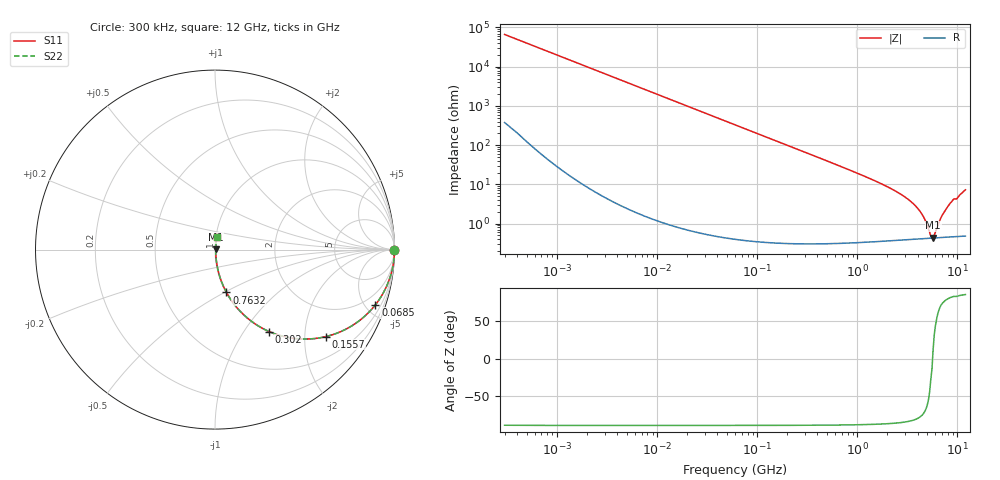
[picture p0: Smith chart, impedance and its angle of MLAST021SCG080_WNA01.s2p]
! MLAST021SCG080_WNA01  S-PARAMETER MODEL  ( General Type )
! Model Generated by TAIYO YUDEN Corporation (http://www.ty-top.com)
! Version 1.0
! TAIYO YUDEN Control No. 220901
! Copyright(c) 2022 TAIYO YUDEN CO.,LTD. All Rights Reserved.
! Product Description (link to TY-COMPAS)
! https://ds.yuden.co.jp/TYCOMPAS/or/detail?pn=MLAST021SCG080CWNA01&u=M
! Products Name : Multilayer Ceramic Capacitors
! Characteristics :
!  Capacitance : 8 pF , Rated Voltage : 25V , TCC : CG / C0G
!  Case Size : 0.25 x 0.125 / 0.0098 x 0.0049 [mm/inch] , Thickness : 0.125 / 0.0049 [mm/inch]
!  (Conditions: Temperature = 25 degC , DC Bias Current/Voltage = 0A / 0V)
! External Node Assignments :
!  1  o---| |---o  2
! GND o---------o GND
! Frequency Range : 0.3MHz  -  12000MHz  [ 401 STEP ]
# MHz S RI R 50
! Freq[MHz].  S11 Real  S11 Imag  S21 Real  S21 Imag  S12 Real  S12 Imag  S22 Real  S22 Imag
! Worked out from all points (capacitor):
!   401 points, 300 kHz to 12 GHz, reference 50 ohm
!   read as one part in series: C = 8 pF near 316.3 kHz
!   lowest |Z| = 440 mohm at 5.715 GHz (marker M1)
!   series resonance near 5.644 GHz, so ESL is about 99 pH
!   S11 on the Smith chart (normalised r, x): 300 kHz: open; 68.5 MHz: 1.01, -5.81; 155.7 MHz: 1.01, -2.55; 302 MHz: 1.01, -1.31; 763.2 MHz: 1.01, -0.51; 12 GHz: 1.01, +0.14
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0.3  1 -0.00151  1.08e-05 0.00151  1.08e-05 0.00151  1 -0.00151
1.769972  0.9999 -0.0089  8.73e-05 0.0089  8.73e-05 0.0089  0.9999 -0.0089
10.44266  0.9972 -0.0523  0.00278 0.0523  0.00278 0.0523  0.9972 -0.0523
27.10171  0.9817 -0.1337  0.0183 0.1337  0.0183 0.1337  0.9817 -0.1337
60  0.9163 -0.2763  0.0837 0.2763  0.0837 0.2763  0.9163 -0.2763
68.49786  0.8937 -0.3076  0.1063 0.3076  0.1063 0.3076  0.8937 -0.3076
101.9188  0.7916 -0.4053  0.2084 0.4053  0.2084 0.4053  0.7916 -0.4053
155.7172  0.6194 -0.4843  0.3806 0.4843  0.3806 0.4843  0.6194 -0.4843
301.9711  0.3023 -0.4569  0.6977 0.4569  0.6977 0.4569  0.3023 -0.4569
353.9943  0.2398 -0.4242  0.7602 0.4242  0.7602 0.4242  0.2398 -0.4242
763.2128  0.064 -0.2387  0.936 0.2387  0.936 0.2387  0.064 -0.2387
2088.533  0.0102 -0.0808  0.9898 0.0808  0.9898 0.0808  0.0102 -0.0808
2947.191  0.00618 -0.0483  0.9938 0.0483  0.9938 0.0483  0.00618 -0.0483
3841.137  0.00475 -0.0271  0.9953 0.0271  0.9953 0.0271  0.00475 -0.0271
4623.766  0.00432 -0.0135  0.9957 0.0135  0.9957 0.0135  0.00432 -0.0135
5420.343  0.00425 -0.00221  0.9958 0.00221  0.9958 0.00221  0.00425 -0.00221
5715.274  0.00428 0.000957  0.9957 -0.000957  0.9957 -0.000957  0.00428 0.000957
6026.253  0.00433 0.00422  0.9957 -0.00422  0.9957 -0.00422  0.00433 0.00422
7064.448  0.00468 0.0158  0.9953 -0.0158  0.9953 -0.0158  0.00468 0.0158
8064.993  0.00526 0.0272  0.9947 -0.0272  0.9947 -0.0272  0.00526 0.0272
8966.534  0.00611 0.0389  0.9939 -0.0389  0.9939 -0.0389  0.00611 0.0389
12000  0.00993 0.0714  0.9901 -0.0714  0.9901 -0.0714  0.00993 0.0714
